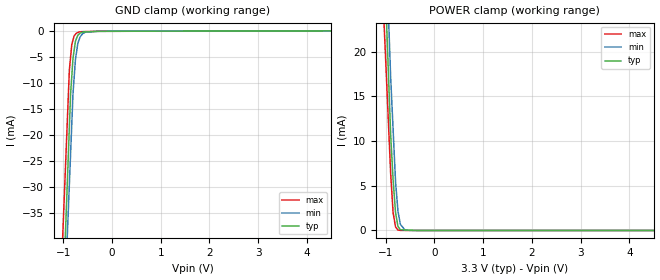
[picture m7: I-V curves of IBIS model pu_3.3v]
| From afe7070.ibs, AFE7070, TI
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[Model] pu_3.3v
Model_type Input
Vinl = 1.00000V
Vinh = 2.30000V
C_comp 562.000fF 550.000fF 574.000fF
| variable typ   min   max
[Voltage Range] 3.30000V 3.00000V 3.60000V
[POWER Clamp Reference] 3.30000V 3.00000V 3.60000V
[GND Clamp Reference] 0.00000V 0.00000V 0.00000V
[Temperature Range] 25   85   -40
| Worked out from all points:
|   GND clamp passes 1 mA (typ) near -0.71 V on its own axis
|   POWER clamp passes 1 mA (typ) near -0.77 V on its own axis
[GND Clamp]
-3.3V     -633.2mA   -595.1mA   -573.9mA
-875mV    -18.46mA   -29.44mA   -7.489mA
-850mV    -12.12mA   -23.61mA   -5.029mA
-825mV    -8.655mA   -17.78mA   -2.57mA
-800mV    -5.19mA    -11.95mA   -1.73mA
-750mV    -1.957mA   -5.47mA    -637.2uA
-725mV    -1.376mA   -3.883mA   -384.8uA
-700mV    -795.2uA   -2.295mA   -297.9uA
-650mV    -398.8uA   -1.068mA   -175.7uA
-600mV    -211.7uA   -498.9uA   -134.6uA
-275mV    -66.46uA   -65.02uA   -68.16uA
6.6V      62.28uA    74.11uA    55.98uA
[POWER Clamp]
-3.3V     368mA      382.7mA    303.9mA
-1.075V   36.81mA    43.83mA    28.1mA
-1.025V   29.36mA    36.22mA    21.9mA
-900mV    10.75mA    17.18mA    6.405mA
-850mV    5.706mA    11.35mA    2.017mA
-800mV    2.016mA    5.509mA    412uA
-750mV    454.9uA    2.158mA    53.54uA
-700mV    76.72uA    675.9uA    9.588uA
-600mV    54.8uA     28.07uA    7.621uA
6.6V      0A         0A         0A
